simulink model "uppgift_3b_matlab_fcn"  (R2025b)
settings: Solver=VariableStepAuto  StartTime=0.0  StopTime=10.0  RelTol=1e-3
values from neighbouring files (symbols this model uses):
  m_dot_end = 14*1e-3    (= 0.014)    [Lektion_2.m]
  m_dot_start = 12*1e-3    (= 0.012)    [Lektion_2.m]
  m_th_1 = 12/1000    (= 0.012)    [Lektion_2.m]
  R = 280    [Lektion_2.m]
  T_i = 320    [Lektion_2.m]
  tau_th = 1/0.1    (= 10)    [Lektion_2.m]
  V_i = 2/1e3    (= 0.002)    [Lektion_2.m]
undefined symbols (not defined in the file or in its folder): p_im

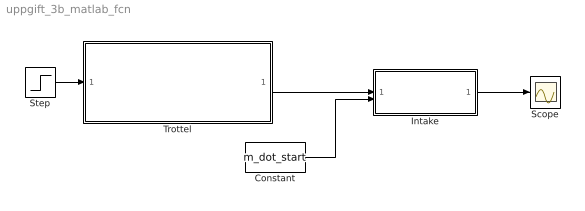
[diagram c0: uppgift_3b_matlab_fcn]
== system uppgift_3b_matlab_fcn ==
  Constant : Constant  Value=m_dot_start
  Intake : Subsystem
  Scope : Scope
  Step : Step  Time=3  Before=m_dot_start  After=m_dot_end  SampleTime=0
  Trottel : Subsystem
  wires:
  Trottel/1(m_at [kg/s]) -> Intake/1(m_at [kg/s])
  Constant/1 -> Intake/2(m_ac [kg/s])
  Intake/1(p_im [Pa]) -> Scope/1
  Step/1 -> Trottel/1(m_at,raf [kg/s])

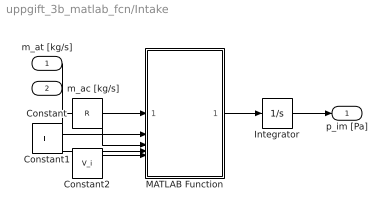
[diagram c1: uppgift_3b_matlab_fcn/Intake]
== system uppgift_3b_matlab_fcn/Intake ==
  m_at [kg/s] : Inport
  m_ac [kg/s] : Inport  Port=2
  Constant : Constant  Value=R
  Constant1 : Constant  Value=T_i
  Constant2 : Constant  Value=V_i
  Integrator : Integrator  InitialCondition=p_im
  MATLAB Function : MATLAB Function  TreatAsAtomicUnit=on
  p_im [Pa] : Outport
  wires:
  Integrator/1 -> p_im [Pa]/1
  MATLAB Function/1(y) -> Integrator/1
  m_ac [kg/s]/1 -> MATLAB Function/2(m_ac)
  m_at [kg/s]/1 -> MATLAB Function/1(m_at)
  Constant/1 -> MATLAB Function/3(R)
  Constant1/1 -> MATLAB Function/4(T)
  Constant2/1 -> MATLAB Function/5(V)

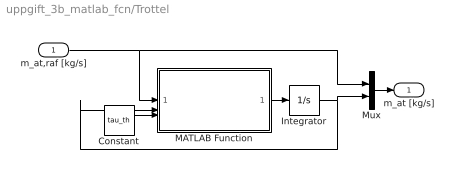
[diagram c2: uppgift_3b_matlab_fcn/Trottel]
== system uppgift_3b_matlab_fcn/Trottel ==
  m_at,raf [kg/s] : Inport
  Constant : Constant  Value=tau_th
  Integrator : Integrator  InitialCondition=m_th_1
  MATLAB Function : MATLAB Function  TreatAsAtomicUnit=on
  Mux : Mux  Inputs=2
  m_at [kg/s] : Outport
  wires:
  Integrator/1 -> MATLAB Function/2(actual), Mux/2
  Mux/1 -> m_at [kg/s]/1
  m_at,raf [kg/s]/1 -> MATLAB Function/1(ref), Mux/1
  MATLAB Function/1(alpha) -> Integrator/1
  Constant/1 -> MATLAB Function/3(tau)

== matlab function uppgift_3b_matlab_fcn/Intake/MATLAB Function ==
function y = fcn(m_at,m_ac,R,T,V)

y = u;

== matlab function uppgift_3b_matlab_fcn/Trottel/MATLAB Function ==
function alpha = fcn(ref, actual, tau)
error = ref - actual;

alpha =  error*tau;
